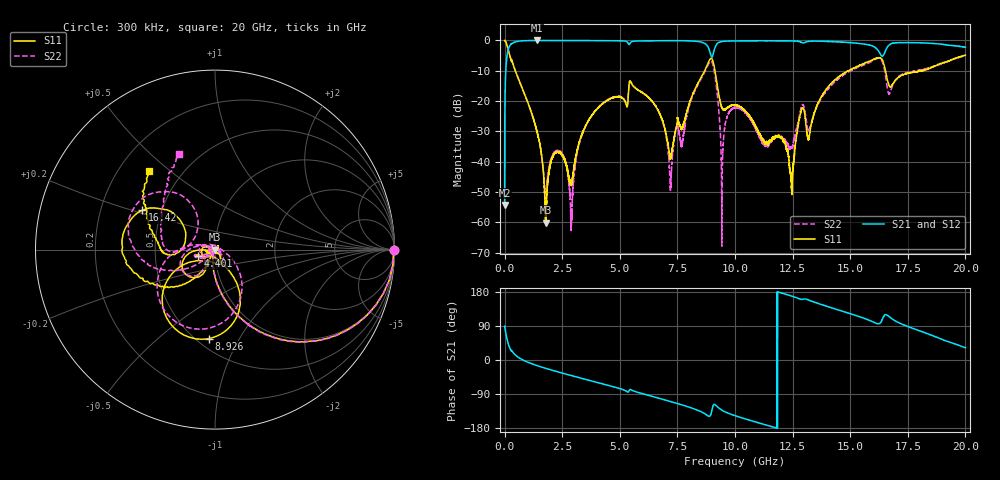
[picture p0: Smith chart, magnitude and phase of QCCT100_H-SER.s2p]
! Created Fri Feb  5 15:28:16 2021
# hz S ma R 50
! 2 Port Network Data from SP1.SP block
! freq  magS11  angS11  magS21  angS21  magS12  angS12  magS22  angS22
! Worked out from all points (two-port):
!   20001 points, 300 kHz to 20 GHz, reference 50 ohm
!   highest |S21| = -0.01 dB at 1.407 GHz (marker M1); lowest = -54.3 dB at 300 kHz (marker M2)
!   |S21| within 3 dB of the highest: 156.9 MHz to 8.879 GHz (8.722 GHz wide, 193 % of centre); 9.102 GHz to 16.18 GHz (7.08 GHz wide, 56 % of centre)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
!   lowest |S11| = -60.1 dB at 1.785 GHz (marker M3), VSWR 1.00, Z = 50.1 - j0.0475 ohm
!   |S11| at or under -10 dB: 465.6 MHz to 8.681 GHz (8.215 GHz wide, 180 % of centre); 9.13 GHz to 14.93 GHz (5.799 GHz wide, 48.2 % of centre); 16.53 GHz to 18.08 GHz (1.548 GHz wide, 8.95 % of centre)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
!   |S22| runs from -67.8 to 0.0 dB; largest |S21 - S12| = 0.017
!   S11 on the Smith chart (normalised r, x): 300 kHz: open; 4.401 GHz: 0.83, -0.06; 8.926 GHz: 0.57, -0.75; 16.42 GHz: 0.39, +0.22; 20 GHz: 0.33, +0.43
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300000  0.9954 -0.2  0.001931 88.9  0.00192 89.9  0.9963 -0.3
1.033e8  0.8321 -34.7  0.5504 55.2  0.5519 55.1  0.8331 -34.7
1.933e8  0.6222 -53.6  0.7796 36.2  0.7798 36.0  0.6238 -53.8
1.4073e9  0.03115 -109.4  0.9994 -14.8  0.9974 -14.8  0.03126 -101.6
1.7853e9  0.0009941 -28.5  0.9984 -22.1  0.9987 -22.1  0.002774 148.9
2.3713e9  0.0141 62.9  0.9966 -32.3  0.9975 -32.4  0.0148 64.6
2.9013e9  0.004147 147.7  0.9977 -41.2  0.9973 -41.1  0.001118 -70.6
3.3343e9  0.02695 -154.8  0.9965 -48.3  0.9966 -48.2  0.02587 -127.3
4.4013e9  0.09965 -158.5  0.9915 -65.4  0.9917 -65.4  0.1015 -151.7
6.6673e9  0.07031 -178.9  0.9908 -100.4  0.9906 -100.4  0.06932 163.7
7.2093e9  0.01175 -100.9  0.9916 -109.6  0.9927 -109.6  0.003755 50.6
7.4483e9  0.03701 -39.5  0.9906 -113.8  0.9907 -113.8  0.0352 -22.1
8.9263e9  0.4975 -94.2  0.6185 -147.2  0.6197 -147.2  0.4537 -102.9
9.4343e9  0.07669 -125.0  0.9588 -132.6  0.9627 -132.6  0.002616 -21.2
1.00003e10  0.08591 -69.6  0.9814 -146.8  0.983 -146.8  0.07791 -54.6
1.20863e10  0.02281 52.1  0.9868 175.6  0.9847 175.7  0.0237 128.4
1.24433e10  0.004806 7.1  0.9821 169.1  0.9818 169.0  0.0169 174.3
1.28773e10  0.0709 -148.2  0.9371 160.1  0.9357 160.1  0.07825 -162.2
1.33343e10  0.04502 -119.2  0.9742 155.0  0.9758 154.9  0.0472 -146.3
1.64153e10  0.4624 151.8  0.5553 110.4  0.5496 110.9  0.4253 130.4
1.66673e10  0.1877 150.5  0.8256 115.4  0.8181 115.7  0.1323 144.4
2e10  0.5708 129.6  0.7724 32.4  0.7615 32.3  0.5693 110.4
